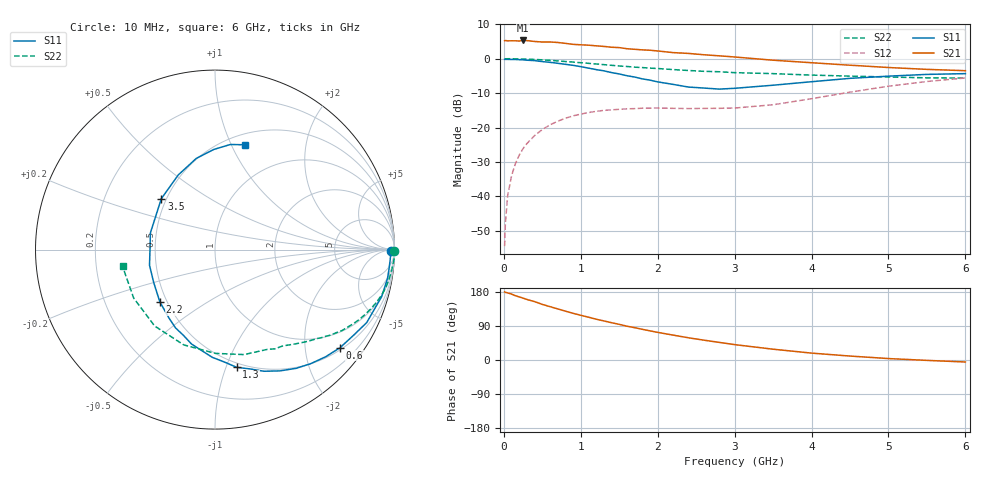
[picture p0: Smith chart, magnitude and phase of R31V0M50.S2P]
! SIEMENS Small Signal Semiconductors
! BFR181
! Si NPN RF Bipolar Junction Transistor in SOT23
! VCE = 1 V  IC = 0.5 mA
! Common Emitter S-Parameters:  May  1996
# GHz  S  MA  R  50
!  f  S11  S21  S12  S22
! GHz  MAG  ANG  MAG  ANG  MAG  ANG  MAG  ANG
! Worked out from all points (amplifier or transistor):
!   36 points, 10 MHz to 6 GHz, reference 50 ohm
!   highest |S21| = 5.3 dB at 250 MHz (marker M1)
!   |S21| within 3 dB of that: start of sweep to 1.976 GHz
!   unconditionally stable (mu >= 1): 2.289 GHz to 4.197 GHz
!   at 250 MHz: K = 0.13, MSG = 15.7 dB, |S12| = -26.1 dB
!   at 1.4 GHz: K = 0.64, MSG = 9.1 dB, |S12| = -14.8 dB
!   at 6 GHz: K = 0.96, MSG = 1.1 dB, |S12| = -5.6 dB
!   S11 on the Smith chart (normalised r, x): 10 MHz: 74, -36; 600 MHz: 0.55, -2.80; 1.3 GHz: 0.46, -1.09; 2.2 GHz: 0.46, -0.33; 3.5 GHz: 0.47, +0.32; 6 GHz: 0.61, +1.13
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0.01  0.9784 -0.6  1.823 179.8  0.0019 93.1  0.9999 -0.3
0.02  0.9787 -1.5  1.835 178.6  0.0041 90.6  0.9958 -0.7
0.05  0.978 -3.1  1.815 177.0  0.0103 90.0  0.9988 -1.6
0.1  0.9756 -6.4  1.82 173.9  0.0199 86.6  0.999 -3.1
0.15  0.9746 -9.5  1.818 169.6  0.0299 82.5  0.9943 -4.8
0.25  0.9647 -15.8  1.84 163.3  0.0496 78.3  0.9886 -7.8
0.4  0.9379 -25.7  1.778 154.1  0.0766 72.3  0.9755 -12.4
0.6  0.8855 -38.1  1.75 140.8  0.1096 63.9  0.9456 -18.2
0.8  0.8291 -50.1  1.67 128.9  0.1366 56.2  0.91 -23.5
1.1  0.7305 -68.1  1.572 113.0  0.1653 46.8  0.8568 -30.2
1.3  0.6667 -79.6  1.508 103.1  0.1776 41.4  0.8201 -34.3
1.5  0.6006 -91.4  1.449 94.1  0.1841 37.2  0.7842 -38.0
1.8  0.5095 -110.1  1.343 81.0  0.1912 32.8  0.7431 -42.5
2.2  0.4238 -136.4  1.226 65.7  0.1903 30.0  0.6955 -48.8
2.4  0.3876 -151.8  1.193 58.6  0.1889 30.2  0.6743 -51.9
2.8  0.3619 178.8  1.101 46.5  0.1905 32.5  0.6466 -58.7
3.5  0.4122 136.5  0.951 28.5  0.2145 41.3  0.607 -74.5
4  0.4635 116.2  0.874 18.2  0.2626 45.8  0.5782 -89.8
4.5  0.5187 101.6  0.805 10.4  0.327 44.8  0.5587 -108.2
5  0.558 90.7  0.745 3.8  0.3987 40.1  0.5424 -128.3
5.5  0.5918 81.7  0.7 -1.0  0.4668 32.8  0.5275 -149.2
6  0.6072 74.1  0.67 -5.3  0.5248 24.4  0.5235 -169.8
